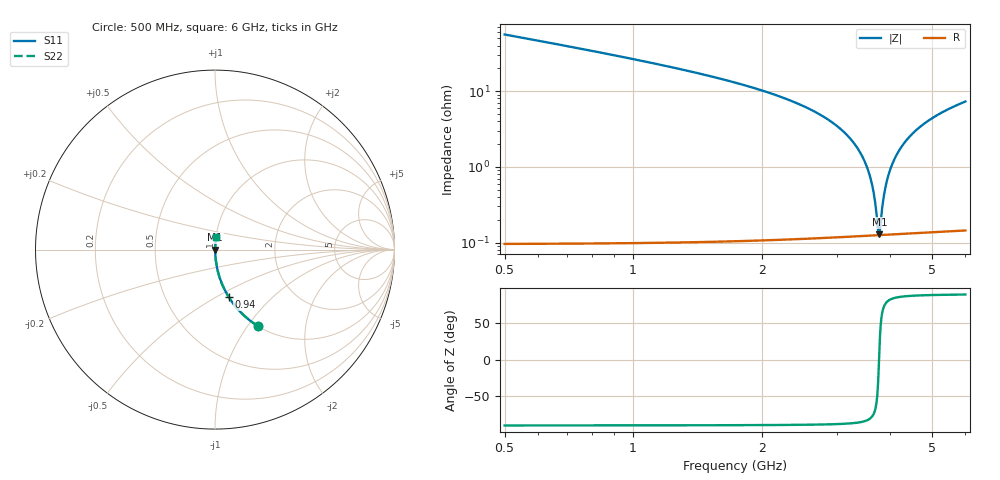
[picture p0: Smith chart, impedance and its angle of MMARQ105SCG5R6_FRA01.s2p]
! MMARQ105SCG5R6_FRA01  S-PARAMETER MODEL  ( General Type )
! Model Generated by TAIYO YUDEN Corporation (http://www.ty-top.com)
! Version 1.0
! TAIYO YUDEN Control No. 200326
! Copyright(c) 2020 TAIYO YUDEN CO.,LTD. All Rights Reserved.
! Product Description (link to TY-COMPAS)
! https://ds.yuden.co.jp/TYCOMPAS/or/detail?pn=MMARQ105SCG5R6CFRA01&u=M
! Products Name : Multilayer Ceramic Capacitors
! Characteristics :
!  Capacitance : 5.6 pF , Rated Voltage : 250V , TCC : CG / C0G
!  Case Size : 1.0 x 0.5 / 0.039 x 0.02 [mm/inch] , Thickness : 0.5 / 0.02 [mm/inch]
!  (Conditions: Temperature = 25 degC , DC Bias Current/Voltage = 0A / 0V)
! External Node Assignments :
!  1  o---| |---o  2
! GND o---------o GND
! Frequency Range : 500MHz  -  6GHz  [ 401 STEP ]
# MHz S RI R 50
! Freq[MHz].  S11 Real  S11 Imag  S21 Real  S21 Imag  S12 Real  S12 Imag  S22 Real  S22 Imag
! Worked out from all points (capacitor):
!   401 points, 500 MHz to 6 GHz, reference 50 ohm
!   read as one part in series: C = 5.58 pF near 527.5 MHz
!   lowest |Z| = 128 mohm at 3.772 GHz (marker M1)
!   series resonance near 3.766 GHz, so ESL is about 320 pH
!   S11 on the Smith chart (normalised r, x): 500 MHz: 1.00, -1.12; 940 MHz: 1.00, -0.57; 6 GHz: 1.00, +0.15
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500  0.2393 -0.4258  0.7607 0.4258  0.7607 0.4258  0.2393 -0.4258
692.5  0.1373 -0.3429  0.8627 0.3429  0.8627 0.3429  0.1373 -0.3429
940  0.0756 -0.2627  0.9244 0.2627  0.9244 0.2627  0.0756 -0.2627
1421.25  0.0297 -0.1667  0.9703 0.1667  0.9703 0.1667  0.0297 -0.1667
2342.5  0.00661 -0.074  0.9934 0.074  0.9934 0.074  0.00661 -0.074
2878.75  0.00284 -0.041  0.9972 0.041  0.9972 0.041  0.00284 -0.041
3250  0.00169 -0.0223  0.9983 0.0223  0.9983 0.0223  0.00169 -0.0223
3428.75  0.00142 -0.0142  0.9986 0.0142  0.9986 0.0142  0.00142 -0.0142
3566.25  0.0013 -0.00823  0.9987 0.00823  0.9987 0.00823  0.0013 -0.00823
3648.75  0.00126 -0.00478  0.9987 0.00478  0.9987 0.00478  0.00126 -0.00478
3690  0.00125 -0.00308  0.9987 0.00308  0.9987 0.00308  0.00125 -0.00308
3745  0.00125 -0.000849  0.9988 0.000849  0.9988 0.000849  0.00125 -0.000849
3772.5  0.00125 0.000254  0.9987 -0.000254  0.9987 -0.000254  0.00125 0.000254
3800  0.00125 0.00135  0.9987 -0.00135  0.9987 -0.00135  0.00125 0.00135
3855  0.00127 0.00352  0.9987 -0.00352  0.9987 -0.00352  0.00127 0.00352
3923.75  0.0013 0.00618  0.9987 -0.00618  0.9987 -0.00618  0.0013 0.00618
4033.75  0.00138 0.0104  0.9986 -0.0104  0.9986 -0.0104  0.00138 0.0104
4171.25  0.00153 0.0154  0.9985 -0.0154  0.9985 -0.0154  0.00153 0.0154
4336.25  0.00176 0.0213  0.9982 -0.0213  0.9982 -0.0213  0.00176 0.0213
4542.5  0.00213 0.0284  0.9979 -0.0284  0.9979 -0.0284  0.00213 0.0284
5092.5  0.0035 0.046  0.9965 -0.046  0.9965 -0.046  0.0035 0.046
6000  0.0067 0.0723  0.9933 -0.0723  0.9933 -0.0723  0.0067 0.0723
